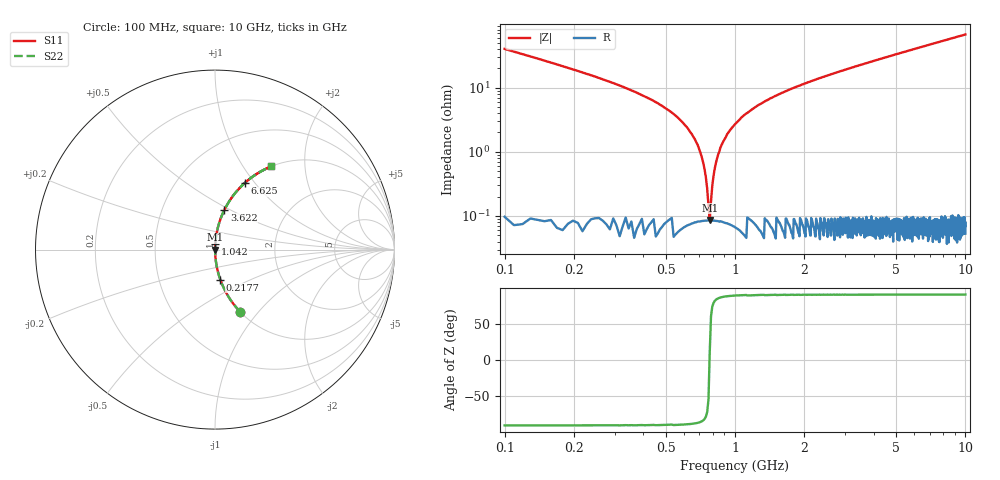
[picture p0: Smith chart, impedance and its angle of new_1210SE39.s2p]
!	AVX	Thin	Film	Operation	Date:	April 2007
!	Description:	Accu-P®	"Series,"	Thin	"Film,"	"SMD,"	RF	Capacitor
!	Part	Number:	12101J390FBT
!	100	MHz	-	5.05	GHz
!	Serial	Measurements
#	MHZ	S	MA	R	50
!	S11	S21	S12	S22
!	dB	Phase	dB	Phase	dB	Phase	dB	Phase
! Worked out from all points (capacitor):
!   1010 points, 100 MHz to 10 GHz, reference 50 ohm
!   read as one part in series: C = 39 pF near 149.1 MHz
!   lowest |Z| = 86.7 mohm at 777 MHz (marker M1)
!   series resonance near 775.8 MHz, so ESL is about 1.1 nH
!   S11 on the Smith chart (normalised r, x): 100 MHz: 1.00, -0.80; 217.7 MHz: 1.00, -0.35; 1.042 GHz: 1.00, +0.06; 3.622 GHz: 1.00, +0.47; 6.625 GHz: 1.00, +0.89; 10 GHz: 1.00, +1.35
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100  0.372 -68.0  0.927 21.9  0.927 21.9  0.372 -68.0
217.74  0.17 -80.0  0.985 9.8  0.985 9.8  0.17 -80.0
512.091  0.045 -86.5  0.998 2.6  0.998 2.6  0.045 -86.5
600.396  0.027 -87.0  0.999 1.6  0.999 1.6  0.027 -87.0
678.89  0.014 -86.3  0.999 0.8  0.999 0.8  0.014 -86.3
708.325  0.0096 -85.3  0.999 0.5  0.999 0.5  0.0096 -85.3
737.76  0.00533 -82.2  0.999 0.3  0.999 0.3  0.00533 -82.2
777.007  0.00072 13.5  0.999 -0.0  0.999 -0.0  0.00072 13.5
806.442  0.00414 80.0  0.999 -0.2  0.999 -0.2  0.00414 80.0
855.5  0.01 85.5  0.999 -0.6  0.999 -0.6  0.01 85.5
894.747  0.015 86.5  0.999 -0.9  0.999 -0.9  0.015 86.5
1041.923  0.031 86.9  0.999 -1.8  0.999 -1.8  0.031 86.9
1316.65  0.058 86.0  0.998 -3.3  0.998 -3.3  0.058 86.0
1758.176  0.096 84.1  0.995 -5.5  0.995 -5.5  0.096 84.1
2454.807  0.148 81.2  0.988 -8.5  0.988 -8.5  0.148 81.2
3406.541  0.214 77.5  0.976 -12.3  0.976 -12.3  0.214 77.5
3622.398  0.228 76.6  0.973 -13.2  0.973 -13.2  0.228 76.6
5054.906  0.317 71.4  0.948 -18.5  0.948 -18.5  0.317 71.4
6624.777  0.405 66.0  0.914 -23.9  0.914 -23.9  0.405 66.0
6703.271  0.409 65.8  0.912 -24.1  0.912 -24.1  0.409 65.8
8351.635  0.489 60.6  0.872 -29.3  0.872 -29.3  0.489 60.6
10000  0.559 56.0  0.829 -34.0  0.829 -34.0  0.559 56.0
